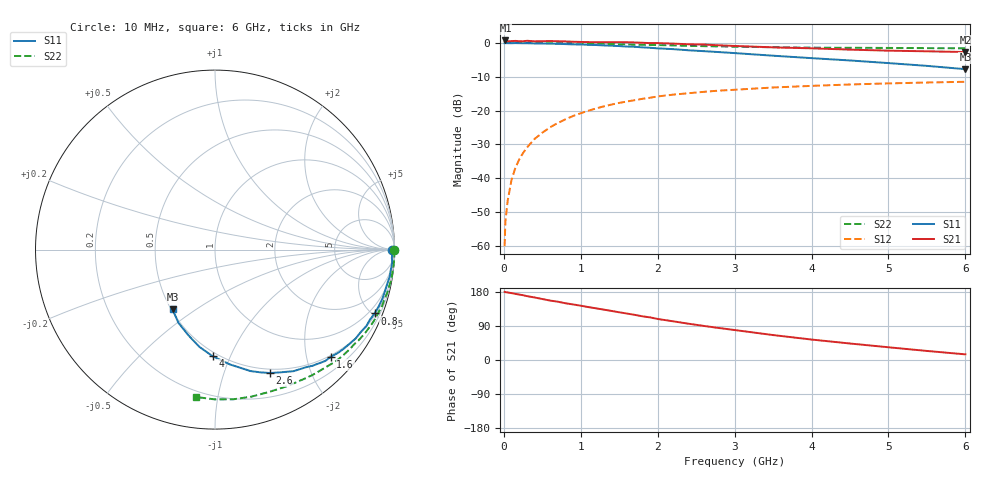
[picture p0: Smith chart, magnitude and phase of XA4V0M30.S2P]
! SIEMENS Discrete & RF Semiconductors
! BFY180
! Si NPN RF Bipolar Junction Transistor in MICRO-X
! VCE = 4 V  IC = 0.3 mA
! Common Emitter S-Parameters:  May  1997
# GHz  S  MA  R  50
!  f  S11  S21  S12  S22
! GHz  MAG  ANG  MAG  ANG  MAG  ANG  MAG  ANG
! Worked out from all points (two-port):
!   36 points, 10 MHz to 6 GHz, reference 50 ohm
!   highest |S21| = 0.69 dB at 20 MHz (marker M1); lowest = -2.7 dB at 6 GHz (marker M2)
!   |S21| within 3 dB of the highest: start of sweep to 4.987 GHz
!   lowest |S11| = -7.8 dB at 6 GHz (marker M3), VSWR 2.38, Z = 25.4 - j20.3 ohm
!   |S11| at or under -10 dB: nowhere
!   |S22| runs from -1.6 to 0.0 dB; largest |S21 - S12| = 1.1
!   S11 on the Smith chart (normalised r, x): 10 MHz: open; 800 MHz: 0.60, -5.13; 1.6 GHz: 0.47, -2.47; 2.6 GHz: 0.45, -1.44; 4 GHz: 0.47, -0.86; 6 GHz: 0.51, -0.41
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0.01  0.9883 -0.2  1.047 179.9  0.001 94.6  0.9989 -0.2
0.02  0.9885 -0.5  1.083 179.0  0.0023 80.6  0.9999 -0.5
0.05  0.9878 -1.4  1.057 178.3  0.0047 87.4  0.9992 -1.0
0.1  0.9864 -2.7  1.059 176.4  0.0095 91.8  0.9999 -2.1
0.15  0.9904 -4.1  1.067 174.5  0.0143 87.1  0.9999 -3.1
0.2  0.988 -5.3  1.056 172.7  0.019 86.1  0.9988 -4.2
0.3  0.986 -8.2  1.071 168.6  0.0285 83.4  0.9969 -6.3
0.4  0.979 -10.9  1.053 165.0  0.0382 81.1  0.9968 -8.3
0.6  0.9719 -16.3  1.061 156.9  0.0566 76.5  0.9909 -12.4
0.8  0.9575 -21.8  1.047 149.8  0.0741 72.1  0.9841 -16.5
1.1  0.933 -29.5  1.024 139.6  0.0997 64.9  0.9734 -22.5
1.3  0.9149 -35.1  1.02 132.9  0.1155 60.6  0.9633 -26.5
1.6  0.8793 -42.8  1.02 122.6  0.1362 54.6  0.946 -32.4
2  0.8278 -52.4  0.99 108.3  0.1618 46.9  0.9261 -39.4
2.2  0.8066 -57.1  0.974 102.1  0.1718 43.1  0.9157 -43.0
2.6  0.7528 -66.0  0.944 89.9  0.1891 36.6  0.8923 -49.3
3  0.7051 -73.7  0.899 79.1  0.203 30.5  0.875 -55.4
3.5  0.6452 -82.6  0.857 65.8  0.2192 24.2  0.8601 -62.3
4  0.5941 -91.3  0.829 54.0  0.2315 18.0  0.8485 -69.1
4.5  0.5488 -99.1  0.793 43.5  0.2429 12.4  0.8439 -76.1
5.5  0.4568 -116.4  0.749 23.9  0.2595 1.8  0.8344 -90.2
6  0.4083 -125.4  0.731 14.9  0.2661 -3.8  0.8278 -97.3
